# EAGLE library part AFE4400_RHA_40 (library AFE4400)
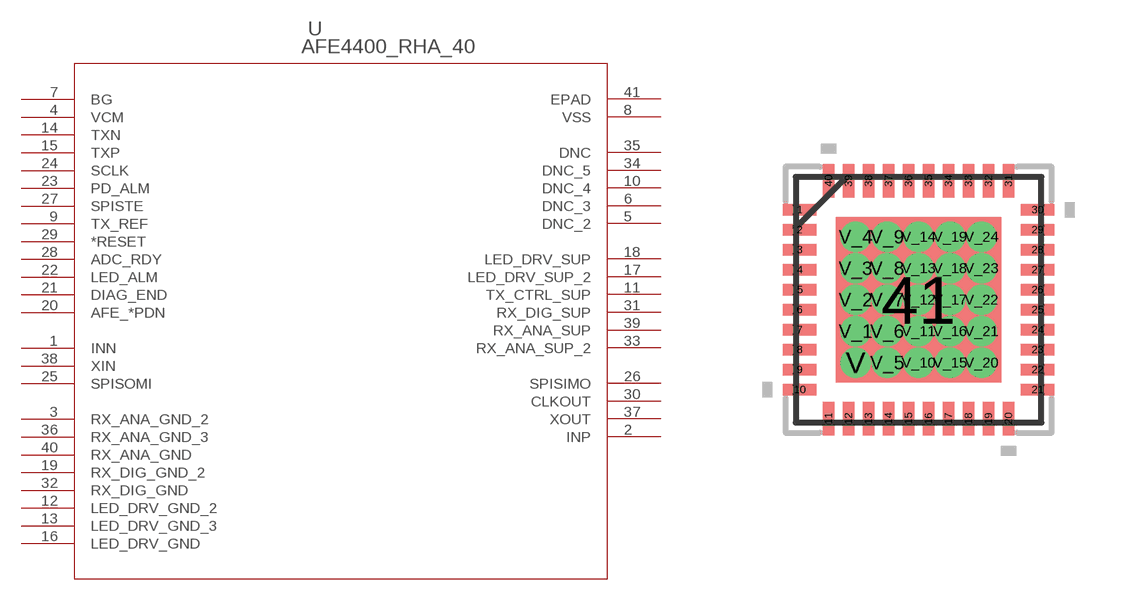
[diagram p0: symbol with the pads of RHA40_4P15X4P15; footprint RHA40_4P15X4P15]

Designator prefix U

## AFE4400_RHA_40 (MANUFACTURER_PART_NUMBER: afe4400_rha_40; VENDOR: Texas Instruments)  [RHA40_4P15X4P15]
1  INN  in
2  INP  in
3  RX_ANA_GND_2  pwr
4  VCM  in
5  DNC_2  nc
6  DNC_3  nc
7  BG  pas
8  VSS  pwr
9  TX_REF  pas
10  DNC_4  nc
11  TX_CTRL_SUP  pas
12  LED_DRV_GND_2  pas
13  LED_DRV_GND_3  pas
14  TXN  out
15  TXP  out
16  LED_DRV_GND  pas
17  LED_DRV_SUP_2  pas
18  LED_DRV_SUP  pas
19  RX_DIG_GND_2  pas
20  AFE_*PDN  in
21  DIAG_END  out
22  LED_ALM  out
23  PD_ALM  out
24  SCLK  pas
25  SPISOMI  in
26  SPISIMO  out
27  SPISTE  pas
28  ADC_RDY  out
29  *RESET  in
30  CLKOUT  out
31  RX_DIG_SUP  pas
32  RX_DIG_GND  pas
33  RX_ANA_SUP_2  pas
34  DNC_5  nc
35  DNC  nc
36  RX_ANA_GND_3  pas
37  XOUT  out
38  XIN  in
39  RX_ANA_SUP  pas
40  RX_ANA_GND  pas
41  EPAD  pas

## Footprint RHA40_4P15X4P15 (pad centres in mm)
smd 0.838 x 0.279: 1 -2.975,2.25; 2 -2.975,1.75; 3 -2.975,1.25; 4 -2.975,0.75; 5 -2.975,0.25; 6 -2.975,-0.25; 7 -2.975,-0.75; 8 -2.975,-1.25; 9 -2.975,-1.75; 10 -2.975,-2.25; 21 2.975,-2.25; 22 2.975,-1.75; 23 2.975,-1.25; 24 2.975,-0.75; 25 2.975,-0.25; 26 2.975,0.25; 27 2.975,0.75; 28 2.975,1.25; 29 2.975,1.75; 30 2.975,2.25
smd 0.279 x 0.838: 11 -2.251,-2.975; 12 -1.75,-2.975; 13 -1.25,-2.975; 14 -0.75,-2.975; 15 -0.25,-2.975; 16 0.25,-2.975; 17 0.75,-2.975; 18 1.25,-2.975; 19 1.75,-2.975; 20 2.251,-2.975; 31 2.251,2.975; 32 1.75,2.975; 33 1.25,2.975; 34 0.75,2.975; 35 0.25,2.975; 36 -0.25,2.975; 37 -0.75,2.975; 38 -1.25,2.975; 39 -1.75,2.975; 40 -2.251,2.975
smd 4.14 x 4.14: 41 0,0
drill 0.254: V -1.575,-1.575; V_1 -1.575,-0.787; V_2 -1.575,0; V_3 -1.575,0.787; V_4 -1.575,1.575; V_5 -0.787,-1.575; V_6 -0.787,-0.787; V_7 -0.787,0; V_8 -0.787,0.787; V_9 -0.787,1.575; V_10 0,-1.575; V_11 0,-0.787; V_12 0,0; V_13 0,0.787; V_14 0,1.575; V_15 0.787,-1.575; V_16 0.787,-0.787; V_17 0.787,0; V_18 0.787,0.787; V_19 0.787,1.575; V_20 1.575,-1.575; V_21 1.575,-0.787; V_22 1.575,0; V_23 1.575,0.787; V_24 1.575,1.575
